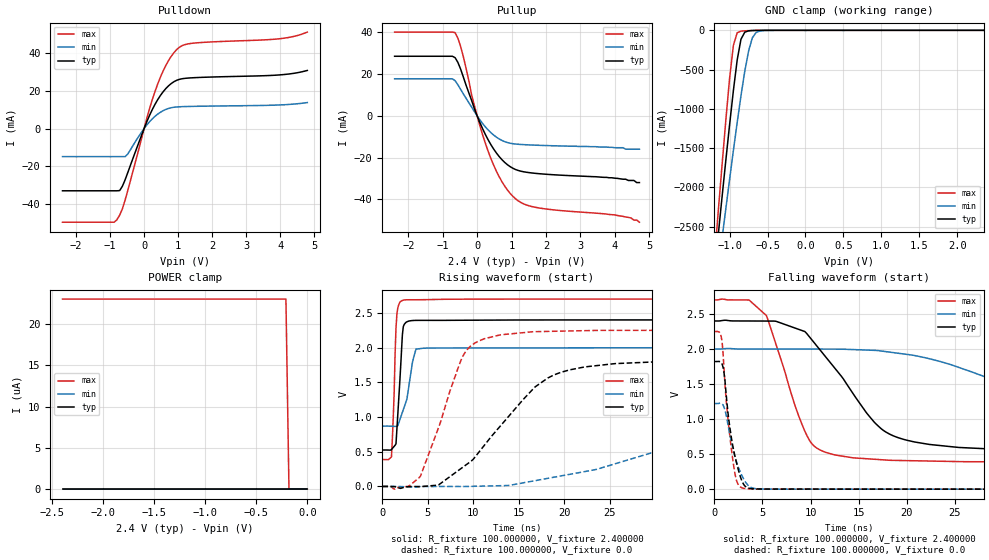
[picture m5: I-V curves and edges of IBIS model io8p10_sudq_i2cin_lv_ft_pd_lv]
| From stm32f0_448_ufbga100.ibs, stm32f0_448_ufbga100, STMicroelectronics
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|   Model io8p10_sudq_i2cin_lv_ft_pd_lv
[Model]  io8p10_sudq_i2cin_lv_ft_pd_lv
Model_type I/O
Polarity   Non-Inverting
Enable   Active-Low
Vinl =   0.720000V
Vinh =   1.680000V
Vmeas =  1.200000V
Cref =   50.000000pF
Rref =   100.000000M
Vref =   0.0V
C_comp   2.067900pF   1.988600pF   2.164800pF
[Temperature Range]   25.000000   0.125000k   -40.000000
[Pullup Reference]   2.400000V   2.000000V   2.700000V
[Pulldown Reference]   0.0V   0.0V   0.0V
[POWER Clamp Reference]   2.400000V   2.000000V   2.700000V
[GND Clamp Reference]   0.0V   0.0V   0.0V
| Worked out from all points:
|   slope of the pulldown table from 0 to 0.36 V, typ, clamps not added: 25.5 ohm
|   slope of the pullup table from 0 to 0.36 V, typ, clamps not added: 28.4 ohm
|   GND clamp passes 1 mA (typ) near -0.64 V on its own axis
|   rising waveform, R_fixture 100.000000, V_fixture 2.400000: 20-80 % time 502ps typ, 1.02ns min, 336ps max; typ from 0.525 V to 2.4 V
|   rising waveform, R_fixture 100.000000, V_fixture 0.0: 20-80 % time 7.29ns typ, 21ns min, 3.54ns max; typ from 0 V to 1.82 V
|   falling waveform, R_fixture 100.000000, V_fixture 2.400000: 20-80 % time 6.29ns typ, 17.2ns min, 3.34ns max; typ from 2.4 V to 0.525 V
|   falling waveform, R_fixture 100.000000, V_fixture 0.0: 20-80 % time 1.17ns typ, 1.36ns min, 921ps max; typ from 1.82 V to 0 V
[Pulldown]
|Voltage   I(typ)   I(min)   I(max)
-2.4V     -33.16mA   -14.98mA   -49.86mA
-880mV    -33.16mA   -14.98mA   -49.86mA
-800mV    -33.16mA   -14.98mA   -48.55mA
-640mV    -30.75mA   -14.98mA   -42.77mA
-480mV    -23.43mA   -13.57mA   -32.92mA
80mV      3.651mA    1.905mA    5.506mA
400mV     15.37mA    7.665mA    23.73mA
720mV     22.75mA    10.69mA    36.23mA
1.04V     26.18mA    11.57mA    43.27mA
1.52V     27.09mA    11.81mA    45.55mA
4V        28.55mA    12.55mA    47.81mA
4.8V      30.9mA     13.81mA    51.31mA
[Pullup]
|Voltage   I(typ)   I(min)   I(max)
-2.4V     28.54mA    17.74mA    40.13mA
-720mV    28.54mA    17.74mA    40.13mA
-640mV    27.85mA    16.83mA    39.87mA
-480mV    22.4mA     12.66mA    33.23mA
-80mV     3.427mA    2.067mA    4.957mA
160mV     -6.219mA   -3.714mA   -9.136mA
320mV     -11.51mA   -6.781mA   -16.98mA
720mV     -21mA      -11.8mA    -31.53mA
1.12V     -25.77mA   -13.54mA   -39.82mA
1.76V     -27.69mA   -14.12mA   -44.06mA
4V        -29.9mA    -15.3mA    -47.5mA
4.72V     -32mA      -16mA      -51mA
[GND_clamp]
|Voltage   I(typ)   I(min)   I(max)
-2.4V     -9.567A    -9.921A    -9.731A
-1.2V     -3.09A     -3.428A    -2.911A
-1.15V    -2.606A    -3.04A     -2.31A
-1.1V     -2.127A    -2.655A    -1.719A
-1.05V    -1.657A    -2.274A    -1.146A
-950mV    -765.3mA   -1.53A     -190.2mA
-900mV    -376.6mA   -1.172A    -30.82mA
-850mV    -112.3mA   -832.5mA   -10.25mA
-750mV    -6.584mA   -264.6mA   -4.043mA
-700mV    -2.596mA   -94.27mA   -2.346mA
-600mV    -430uA     -8.168mA   -383.4uA
2.35V     59.64uA    46.24uA    66.77uA
[POWER_clamp]
|Voltage   I(typ)   I(min)   I(max)
-2.4V     0A         0A         23.03uA
-210mV    0A         0A         23.03uA
-180mV    0A         0A         0A
0V        0A         0A         0A
[Ramp]
| variable   typ   min   max
dV/dt_r  1.09218/7.28034n   0.73200/20.91606n   1.34880/3.53972n
dV/dt_f  1.12426/6.28340n   0.67635/17.47089n   1.38699/3.33715n
R_load = 100.000000
[Rising Waveform]
R_fixture= 100.000000
V_fixture= 2.400000
V_fixture_min= 2.000000
V_fixture_max= 2.700000
|time   V(typ)   V(min)   V(max)
0s        524.8mV    868.7mV    387.2mV
1.001ns   532.7mV    867.1mV    426.3mV
1.301ns   578mV      865.5mV    1.362V
1.401ns   593.1mV    865.2mV    1.916V
1.502ns   615.5mV    864.9mV    2.285V
1.702ns   1.044V     875.3mV    2.573V
2.202ns   2.183V     1.067V     2.679V
2.503ns   2.35V      1.183V     2.687V
3.704ns   2.392V     1.979V     2.689V
49.85ns   2.399V     1.999V     2.699V
[Rising Waveform]
R_fixture= 100.000000
V_fixture= 0.0
V_fixture_min= 0.0
V_fixture_max= 0.0
|time   V(typ)   V(min)   V(max)
0s        1.433nV    15.35nV    1.088nV
2.803ns   -3.389mV   -6.23mV    -1.57mV
4.204ns   -1.791mV   -2.125mV   151.4mV
8.809ns   273mV      -640.2uV   1.865V
10.21ns   426.1mV    2.667mV    2.068V
13.01ns   875.4mV    10.9mV     2.184V
18.22ns   1.563V     117.3mV    2.233V
25.63ns   1.77V      327.1mV    2.248V
51.25ns   1.821V     1.098V     2.248V
99.7ns    1.82V      1.221V     2.248V
[Falling Waveform]
R_fixture= 100.000000
V_fixture= 2.400000
V_fixture_min= 2.000000
V_fixture_max= 2.700000
|time   V(typ)   V(min)   V(max)
0s        2.399V     1.999V     2.699V
3.604ns   2.399V     1.998V     2.698V
5.405ns   2.398V     1.998V     2.476V
9.61ns    2.219V     1.997V     768.1mV
12.61ns   1.711V     1.997V     486.6mV
17.82ns   816.8mV    1.962V     415.8mV
25.43ns   594.9mV    1.737V     393.3mV
31.63ns   554.7mV    1.426V     389.3mV
46.65ns   529.5mV    997.3mV    387.4mV
99.7ns    524.8mV    868.7mV    387.2mV
[Falling Waveform]
R_fixture= 100.000000
V_fixture= 0.0
V_fixture_min= 0.0
V_fixture_max= 0.0
|time   V(typ)   V(min)   V(max)
0s        1.82V      1.221V     2.248V
700.7ps   1.801V     1.221V     2.179V
800.8ps   1.783V     1.214V     2.098V
1.001ns   1.655V     1.164V     1.71V
1.401ns   1.097V     924.9mV    1.009V
1.902ns   622.2mV    594.7mV    429.2mV
2.302ns   373.6mV    386.6mV    122.4mV
2.903ns   103.3mV    181.7mV    16.92mV
4.705ns   2.133mV    3.52mV     1.919mV
49.85ns   1.433nV    15.35nV    1.088nV
